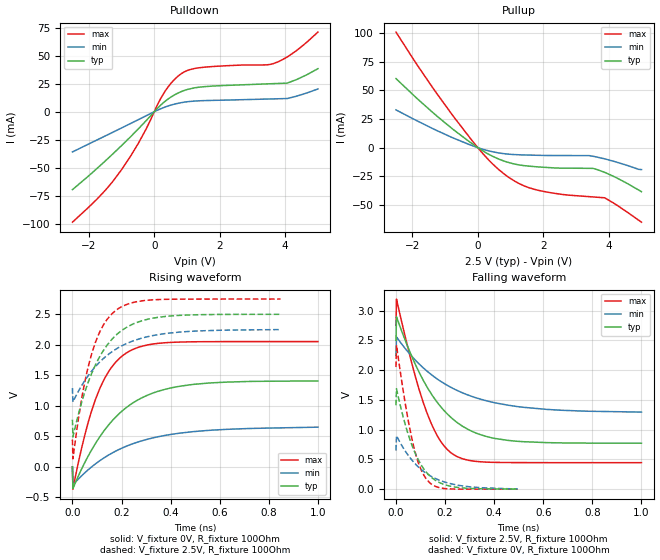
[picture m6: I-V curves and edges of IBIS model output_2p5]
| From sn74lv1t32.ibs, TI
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|   output_2p5 Model
[Model]   output_2p5
Model_type   Output
Polarity   Inverting
Vmeas = 1.25
Vref = 0
Cref = 30pF
Rref = 250
|   typ   min   max
|   (nom PVT)   (fast PVT)   (slow PVT)
C_comp   1.684e-12   1.569e-12   1.775e-12
| Where nom  PVT is Nominal Process, 2.5V, 40C
|   Fast PVT is Strong Process,  2.75V, -40C
|   Slow PVT is Weak Process,   2.25V, 140C
[Voltage Range]   2.5   2.25   2.75
|Junction Temperature
[Temperature Range]   40   140   -40
[Pullup Reference]   2.5   2.25   2.75
[Pulldown Reference]   0   0   0
[Power Clamp Reference]   2.5   2.25   2.75
[GND Clamp Reference]   0   0   0
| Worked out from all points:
|   slope of the pulldown table from 0 to 0.375 V, typ, clamps not added: 36.4 ohm
|   slope of the pullup table from 0 to 0.375 V, typ, clamps not added: 58.5 ohm
|   falling waveform, V_fixture 2.5V, R_fixture 100Ohm: 20-80 % time 177ps typ, 262ps min, 113ps max; typ from 2.5 V to 0.773 V
|   rising waveform, V_fixture 0V, R_fixture 100Ohm: 20-80 % time 202ps typ, 263ps min, 118ps max; typ from 0 V to 1.41 V
|   rising waveform, V_fixture 2.5V, R_fixture 100Ohm: 20-80 % time 135ps typ, 181ps min, 92.3ps max; typ from 0.772 V to 2.5 V
|   falling waveform, V_fixture 0V, R_fixture 100Ohm: 20-80 % time 89.2ps typ, 130ps min, 64.2ps max; typ from 1.41 V to 0.001 V
[Pulldown]
|   Voltage   I(typ)   I(min)   I(max)
-2.5V     -69.62mA   -35.93mA   -98.69mA
-1.488V   -43.76mA   -21.51mA   -69.97mA
-995.8mV  -30.19mA   -14.46mA   -51.61mA
-476mV    -15.02mA   -6.953mA   -27.74mA
313.2mV   8.882mA    3.986mA    17.51mA
569mV     14.18mA    6.391mA    27.33mA
800mV     17.65mA    7.956mA    33.42mA
1.064V    20.28mA    9.098mA    37.4mA
1.357V    21.86mA    9.724mA    39.21mA
3.624V    25.07mA    11.44mA    42.86mA
4.061V    25.55mA    11.77mA    48.85mA
5V        38.44mA    20.33mA    71.13mA
[Pullup]
|   Voltage   I(typ)   I(min)   I(max)
-2.5V     60.3mA     32.97mA    100.9mA
-1.821V   41.99mA    22.91mA    70.85mA
-715.7mV  15.06mA    7.996mA    26.2mA
134.8mV   -2.5mA     -1.243mA   -4.574mA
457.5mV   -7.614mA   -3.621mA   -14.36mA
789.5mV   -11.6mA    -5.221mA   -22.67mA
1.248V    -15.01mA   -6.211mA   -31.16mA
1.744V    -16.58mA   -6.612mA   -36.51mA
2.565V    -17.87mA   -6.888mA   -40.79mA
3.52V     -18.08mA   -7.535mA   -43.03mA
3.872V    -21.54mA   -9.754mA   -43.77mA
5V        -38.46mA   -19.14mA   -65.08mA
[Ramp]
R_load = 100
|   typ   min   max
dV/dt_r   0.844816/2.01731e-10  0.386728/2.57059e-10   1.23182/1.17822e-10
dV/dt_f   1.03649/1.771e-10   0.572674/2.61835e-10   1.38235/1.13243e-10
[Falling Waveform]
V_fixture = 2.5V
V_fixture_min = 2.25V
V_fixture_max = 2.75V
R_fixture = 100Ohm
|   Time   V(typ)   V(min)   V(max)
0s        2.5V       2.25V      2.75V
2ps       2.9V       2.559V     3.195V
72ps      2.16V      2.199V     1.998V
126ps     1.721V     1.985V     1.285V
182ps     1.387V     1.813V     804.9mV
242ps     1.143V     1.673V     562.8mV
334ps     930.3mV    1.525V     463.8mV
456ps     820mV      1.412V     447.6mV
674ps     777.8mV    1.326V     446.1mV
1ns       772.5mV    1.296V     446.1mV
[Rising Waveform]
V_fixture = 0V
V_fixture_min = 0V
V_fixture_max = 0V
R_fixture = 100Ohm
|   Time   V(typ)   V(min)   V(max)
0s        370pV      6.466nV    529.4pV
2ps       -358.3mV   -298.4mV   -367.2mV
34ps      -64.97mV   -162.1mV   246.5mV
64ps      174.3mV    -50.05mV   723.8mV
126ps     574.9mV    139mV      1.408V
176ps     814.6mV    256.1mV    1.714V
238ps     1.025V     365.9mV    1.908V
350ps     1.239V     493.1mV    2.024V
484ps     1.347V     572.7mV    2.049V
1ns       1.408V     649.5mV    2.053V
[Rising Waveform]
V_fixture = 2.5V
V_fixture_min = 2.25V
V_fixture_max = 2.75V
R_fixture = 100Ohm
|   Time   V(typ)   V(min)   V(max)
0s        772.2mV    1.29V      446.1mV
2ps       488.3mV    1.063V     128.2mV
28ps      916.2mV    1.265V     879.7mV
46ps      1.168V     1.385V     1.299V
90ps      1.638V     1.625V     1.997V
130ps     1.93V      1.788V     2.349V
186ps     2.188V     1.95V      2.59V
258ps     2.36V      2.079V     2.704V
378ps     2.465V     2.184V     2.745V
848ps     2.5V       2.249V     2.75V
[Falling Waveform]
V_fixture = 0V
V_fixture_min = 0V
V_fixture_max = 0V
R_fixture = 100Ohm
|   Time   V(typ)   V(min)   V(max)
0s        1.409V     649.7mV    2.053V
2ps       1.688V     899.3mV    2.42V
40ps      1.054V     626.4mV    1.386V
56ps      843.2mV    534.6mV    1.023V
72ps      664.8mV    454.7mV    719.4mV
102ps     411.5mV    333.7mV    329.1mV
138ps     222.2mV    228.5mV    105.8mV
176ps     112.9mV    152.3mV    25.91mV
240ps     35.77mV    76.54mV    2.092mV
496ps     1.216mV    4.821mV    136.2uV
